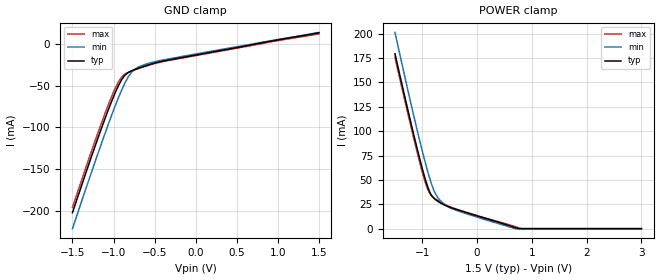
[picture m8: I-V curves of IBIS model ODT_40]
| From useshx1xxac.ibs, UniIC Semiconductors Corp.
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|   Model ODT_40
[Model]  ODT_40
Model_type   Input
Polarity   Non-Inverting
Vinl =   0.600000V
Vinh =   0.900000V
C_comp   1.3900pF   1.3640pF   1.5600pF
[Temperature Range]   25.0000   95.0000   0.0
[Voltage Range]   1.5000V   1.4000V   1.6000V
[GND_clamp]
|Voltage   I(typ)   I(min)   I(max)
-1.5V     -202.2mA   -221.3mA   -195.9mA
-1.18V    -110.1mA   -128.6mA   -103.8mA
-1.06V    -78.08mA   -95.39mA   -72.11mA
-980mV    -58.58mA   -74.39mA   -53.36mA
-940mV    -49.98mA   -64.47mA   -45.55mA
-900mV    -42.75mA   -55.15mA   -39.69mA
-860mV    -37.52mA   -46.7mA    -36.14mA
-780mV    -32.38mA   -34.07mA   -32.57mA
-740mV    -30.83mA   -30.39mA   -31.17mA
-620mV    -26.73mA   -24.85mA   -27.23mA
-420mV    -21.2mA    -19.83mA   -21.79mA
1.5V      13.07mA    13.58mA    11.78mA
[POWER_clamp]
|Voltage   I(typ)   I(min)   I(max)
-1.5V     179.4mA    201.3mA    175.8mA
-1.14V    92.41mA    111.8mA    88.75mA
-1.02V    65.56mA    83.92mA    61.98mA
-940mV    49.42mA    66.45mA    46.34mA
-860mV    36.94mA    50.57mA    35.75mA
-780mV    30.73mA    38.04mA    31.23mA
-700mV    27.46mA    30.62mA    28.33mA
-600mV    24.37mA    25.09mA    25.22mA
-480mV    21.66mA    20.93mA    22.01mA
-240mV    17.27mA    16.15mA    17.56mA
752.8mV   0A         NA         NA
3V        0A         0A         0A
